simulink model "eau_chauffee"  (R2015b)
settings: Solver=ode23t  StartTime=0.0  StopTime=30000  RelTol=1e-3
libraries: fl_lib x4, nesl_utility x3

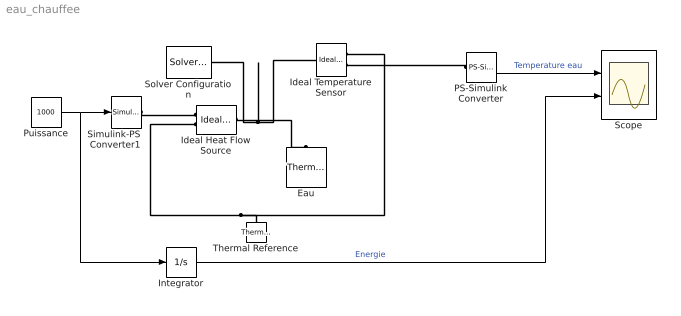
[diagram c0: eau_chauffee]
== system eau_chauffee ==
  Eau : fl_lib/Thermal/Thermal Elements/Thermal Mass  mass=0 kg  sp_heat=0 J/kg/K  Q_specify=off  Q_priority=None  Q=0 J/s  T_specify=on  T_priority=High  T=0 C
  Ideal Heat Flow Source : fl_lib/Thermal/Thermal Sources/Ideal Heat Flow Source
  Ideal Temperature Sensor : fl_lib/Thermal/Thermal Sensors/Ideal Temperature Sensor
  Integrator : Integrator
  PS-Simulink Converter : nesl_utility/PS-Simulink Converter  PhysicalDomain=network_engine_domain  SubClassName=ps_output  LeftPortType=input  RightPortType=output  PseudoPeriodic=off  Frequencies=[]  Unit=C  AffineConversion=on
  Puissance : Constant  Value=1000
  Scope : Scope  NumInputPorts=2
  Simulink-PS Converter1 : nesl_utility/Simulink-PS Converter  PhysicalDomain=network_engine_domain  SubClassName=ps_input  LeftPortType=input  RightPortType=output  PseudoPeriodic=off  Frequencies=[]  NoiseDistribution=none  NoiseParameters=[]  Unit=W  AffineConversion=on  InputFiltering=off  SimscapeFilterOrder=1  InputFilterTimeConstant=.001  UdotUserProvided=0
  Solver Configuration : nesl_utility/Solver Configuration  PhysicalDomain=network_engine_domain  SubClassName=solver  LeftPortType=input  RightPortType=generic  Accelerate=off  Tones=[]  Harmonics=[]  SimulateNoise=off  Profile=off  UseLocalSampling=off  EnableSwitchedLinearOptims=on  FrequencyDomain=off  UseCCode=off  RelTol=0.001  AbsTol=1e-06  MinStep=1e-09  ToWorkspace=off  RevertToSquareIcSolve=off  NumHomotopyIterations=100  PhasorMode=off  PhasorModeNumHarmonics=1  DoDC=off  ResidualTolerance=1e-09  UseLocalSolver=off  LocalSolverChoice=NE_BACKWARD_EULER_ADVANCER  LocalSolverSampleTime=0.001  DoFixedCost=off  MaxNonlinIter=3  MaxModeIter=2  LinearAlgebra=Sparse  DelaysMemoryBudget=1024  AutomaticFiltering=on  FilteringTimeConstant=0.001
  Thermal Reference : fl_lib/Thermal/Thermal Elements/Thermal Reference
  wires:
  Puissance/1 -> Simulink-PS Converter1/1, Integrator/1
  PS-Simulink Converter/1 -> Scope/1  "Temperature eau"
  Integrator/1 -> Scope/2  "Energie"
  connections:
  Ideal Heat Flow Source/LConn1 -- Solver Configuration/RConn1 -- Ideal Temperature Sensor/LConn1 -- Eau/LConn1
  Ideal Temperature Sensor/RConn1 -- Thermal Reference/LConn1 -- Ideal Heat Flow Source/RConn2
  Simulink-PS Converter1/RConn1 -- Ideal Heat Flow Source/RConn1
  PS-Simulink Converter/LConn1 -- Ideal Temperature Sensor/RConn2
